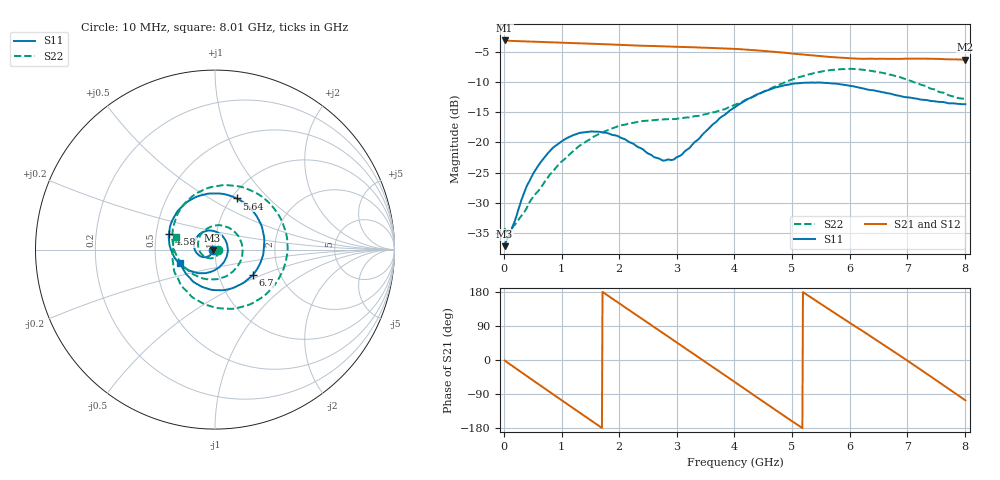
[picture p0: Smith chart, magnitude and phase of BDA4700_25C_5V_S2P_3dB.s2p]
!Agilent Technologies,E5071B,MY42404982,A.09.10
!Date: Mon Oct 20 13:27:23 2025
!Data & Calibration Information:
!Freq	S11:SOLT2(ON)	S21:SOLT2(ON)	S12:SOLT2(ON)	S22:SOLT2(ON)
# Hz S RI R 50
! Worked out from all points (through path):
!   801 points, 10 MHz to 8.01 GHz, reference 50 ohm
!   highest |S21| = -3.11 dB at 10 MHz (marker M1); lowest = -6.3 dB at 8.01 GHz (marker M2)
!   group delay of S21, straight-line fit = 286 ps
!   lowest |S11| = -37.2 dB at 10 MHz (marker M3), VSWR 1.03, Z = 48.6 - j0.161 ohm
!   |S11| at or under -10 dB: start of sweep to end of sweep
!   |S22| runs from -34.8 to -7.8 dB; largest |S21 - S12| = 0.0051
!   S11 on the Smith chart (normalised r, x): 10 MHz: 0.97, -0.00; 4.58 GHz: 0.58, +0.11; 5.64 GHz: 1.06, +0.67; 6.7 GHz: 1.46, -0.44; 8.01 GHz: 0.67, -0.10
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1e7  -0.0138 -0.00166  0.6986 -0.0147  0.6988 -0.0158  0.0194 -0.00185
3.3e8  -0.0237 -0.0275  0.5607 -0.3989  0.5604 -0.3996  0.0177 -0.0185
7.2e8  -0.0649 -0.0416  0.1567 -0.6603  0.1568 -0.6603  -0.0117 -0.0469
1.02e9  -0.1019 -0.0193  -0.2094 -0.6374  -0.2096 -0.6376  -0.0588 -0.0392
1.35e9  -0.1163 0.0322  -0.5274 -0.4005  -0.5275 -0.4006  -0.0943 0.0203
1.64e9  -0.0938 0.0792  -0.6487 -0.0786  -0.6491 -0.0785  -0.0739 0.0906
1.93e9  -0.0458 0.105  -0.5925 0.2545  -0.5925 0.2553  -0.00105 0.1334
2.32e9  0.0259 0.088  -0.2821 0.568  -0.282 0.5681  0.1133 0.0951
2.68e9  0.0669 0.0311  0.1159 0.6155  0.1164 0.6156  0.1533 -0.0183
3.36e9  0.0151 -0.1036  0.6043 0.0965  0.6048 0.0959  -0.0014 -0.1656
3.67e9  -0.0647 -0.1315  0.5554 -0.2372  0.5553 -0.2388  -0.1029 -0.1462
4.01e9  -0.1672 -0.1029  0.3095 -0.5073  0.31 -0.5072  -0.1914 -0.073
4.58e9  -0.2565 0.0871  -0.2679 -0.5013  -0.2679 -0.502  -0.2254 0.152
4.97e9  -0.1819 0.2424  -0.5076 -0.2021  -0.5085 -0.2029  -0.1085 0.3097
5.35e9  -0.0182 0.3128  -0.5028 0.1531  -0.5035 0.1523  0.1071 0.3552
5.64e9  0.1218 0.2851  -0.3554 0.3672  -0.3553 0.3678  0.2746 0.2839
6.14e9  0.2677 0.1004  0.0466 0.4923  0.0492 0.4928  0.4042 -0.00968
6.68e9  0.2166 -0.1343  0.4221 0.2529  0.4233 0.2518  0.2237 -0.2904
6.7e9  0.2115 -0.1407  0.431 0.2373  0.4314 0.2367  0.2125 -0.2963
7.26e9  0.00408 -0.2258  0.4355 -0.2338  0.4355 -0.2346  -0.1014 -0.2808
7.64e9  -0.1239 -0.1764  0.1848 -0.4527  0.1842 -0.454  -0.2278 -0.12
8.01e9  -0.1938 -0.0742  -0.1374 -0.4637  -0.1371 -0.4644  -0.2187 0.0698
